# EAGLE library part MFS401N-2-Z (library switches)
4PDT Switch
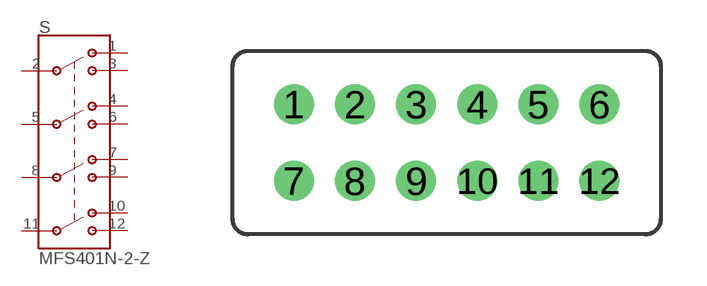
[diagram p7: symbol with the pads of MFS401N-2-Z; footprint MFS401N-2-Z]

Designator prefix S

## MFS401N-2-Z (DIGIKEY: 563-1568-ND)  [MFS401N-2-Z]
1  1TA
2  1P
3  1TB
4  2TA
5  2P
6  2TB
7  3TA
8  3P
9  3TB
10  4TA
11  4P
12  4TB

## Footprint MFS401N-2-Z (pad centres in mm)
Copal Electronics 4PDT http://www.nidec-copal-electronics.com/e/catalog/switch/mfs.pdf
drill 0.8: 1 -5,1.25; 2 -3,1.25; 3 -1,1.25; 4 1,1.25; 5 3,1.25; 6 5,1.25; 7 -5,-1.25; 8 -3,-1.25; 9 -1,-1.25; 10 1,-1.25; 11 3,-1.25; 12 5,-1.25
